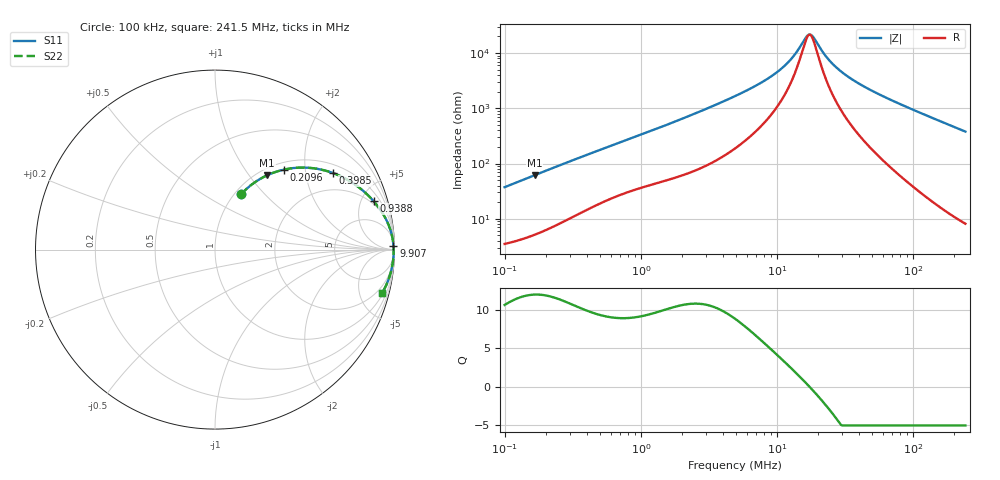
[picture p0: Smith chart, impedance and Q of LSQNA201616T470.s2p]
! LSQNA201616T470  S-PARAMETER MODEL  ( General Type )
! Model Generated by TAIYO YUDEN Corporation (http://www.ty-top.com)
! Version 2.0
! TAIYO YUDEN Control No. 100810NF25SB-FKC
! Copyright(c) 2007 TAIYO YUDEN CO.,LTD. All Rights Reserved.
! Product Description (link to TY-COMPAS)
! https://ds.yuden.co.jp/TYCOMPAS/or/detail?pn=LSQNA201616T470K&u=M
! Products Name : Inductors
! Characteristics :
!  Inductance : 47 uH , SRF(min) : 11 MHz , DC Resistance(max) : 3.12 Ohm
!  Rated Current : Saturation :110 mA , Temp Rise : 240 mA (40 degC)
!  Case Size : 2.0 x 1.6 / 0.079 x 0.063 [mm/inch] , Thickness : 1.6 / 0.063 [mm/inch]
!  (Conditions: Temperature = 25 degC , DC Bias Current/Voltage = 0A / 0V)
! External Node Assignments :
!  1  o---GGG---o  2
! GND o---------o GND
! Frequency Range : 0.1MHz  -  241.513628MHz  [ 402 STEP ]
# MHz S RI R 50
! Freq[MHz].  S11 Real  S11 Imag  S21 Real  S21 Imag  S12 Real  S12 Imag  S22 Real  S22 Imag
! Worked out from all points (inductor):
!   401 points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, 100 kHz to 241.5 MHz, reference 50 ohm
!   read as one part in series: L = 59 uH near 104 kHz
!   highest Q = 11.9 at 165.9 kHz (marker M1), where L = 58.8 uH
!   self-resonance near 17.09 MHz
!   S11 on the Smith chart (normalised r, x): 100 kHz: 1.07, +0.74; 209.6 kHz: 1.13, +1.54; 398.5 kHz: 1.29, +2.84; 938.8 kHz: 1.69, +6.23; 9.907 MHz: 21, +86; 241.5 MHz: 1.16, -7.57
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0.1  0.1442 0.3072  0.8558 -0.3072  0.8558 -0.3072  0.1442 0.3072
0.165917  0.2899 0.4137  0.7101 -0.4137  0.7101 -0.4137  0.2899 0.4137
0.209594  0.3832 0.4455  0.6168 -0.4455  0.6168 -0.4455  0.3832 0.4455
0.368674  0.6256 0.4371  0.3744 -0.4371  0.3744 -0.4371  0.6256 0.4371
0.39854  0.6558 0.4272  0.3442 -0.4272  0.3442 -0.4272  0.6558 0.4272
0.599897  0.7876 0.3572  0.2124 -0.3572  0.2124 -0.3572  0.7876 0.3572
0.938849  0.8832 0.2706  0.1168 -0.2706  0.1168 -0.2706  0.8832 0.2706
1.359207  0.9325 0.2048  0.0675 -0.2048  0.0675 -0.2048  0.9325 0.2048
2.687156  0.9768 0.1111  0.0232 -0.1111  0.0232 -0.1111  0.9768 0.1111
4.914404  0.9897 0.0589  0.0103 -0.0589  0.0103 -0.0589  0.9897 0.0589
7.397334  0.9931 0.0352  0.00692 -0.0352  0.00692 -0.0352  0.9931 0.0352
9.90685  0.9943 0.0217  0.00567 -0.0217  0.00567 -0.0217  0.9943 0.0217
12.7609  0.995 0.0115  0.00502 -0.0115  0.00502 -0.0115  0.995 0.0115
16.43716  0.9954 0.00199  0.00464 -0.00199  0.00464 -0.00199  0.9954 0.00199
17.42604  0.9954 -0.000189  0.00459 0.000189  0.00459 0.000189  0.9954 -0.000189
18.11814  0.9954 -0.00164  0.00456 0.00164  0.00456 0.00164  0.9954 -0.00164
23.33776  0.9955 -0.0113  0.00451 0.0113  0.00451 0.0113  0.9955 -0.0113
29.48135  0.9953 -0.0209  0.0047 0.0209  0.0047 0.0209  0.9953 -0.0209
41.05087  0.9945 -0.0366  0.00551 0.0366  0.00551 0.0366  0.9945 -0.0366
66.79689  0.9912 -0.0675  0.00875 0.0675  0.00875 0.0675  0.9912 -0.0675
129.5109  0.9766 -0.1359  0.0234 0.1359  0.0234 0.1359  0.9766 -0.1359
241.5136  0.9302 -0.2443  0.0698 0.2443  0.0698 0.2443  0.9302 -0.2443
